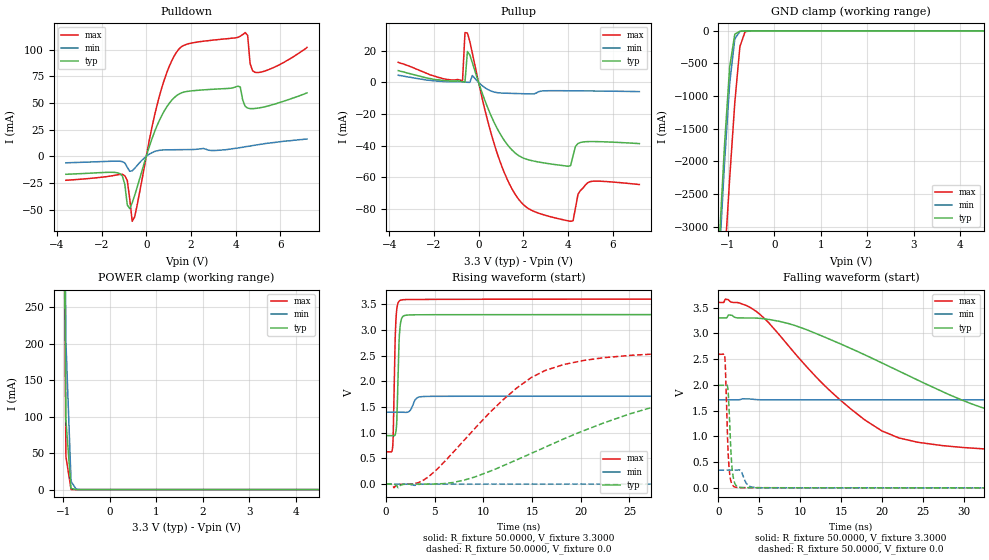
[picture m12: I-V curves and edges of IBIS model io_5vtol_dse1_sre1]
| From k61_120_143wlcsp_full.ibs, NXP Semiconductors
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[Model]  io_5vtol_dse1_sre1
|   Model io_5vtol_dse1_sre1
| Library cells for typ/min/max conditions are connected as defined below:
|  pad - External Pad
|  ipp_do - Core Input
|  ipp_obe - Output Buffer Enable
|  esd_boost - vdd_s_3v
|  esd_bus - vdd_s_3v
|  ipp_ame - vss_s_lv
|  ipp_dse - vdd_s_lv
|  ipp_ina40a_5vtol - NC
|  ipp_ina40b_5vtol - NC
|  ipp_ina_5vtol - NC
|  ipp_ina_mux_3v - NC
|  ipp_ind - NC
|  ipp_ind_3v - NC
|  ipp_pue - vss_s_lv
|  ipp_sre - vdd_s_lv
|  tie_3v - vdd_s_3v
|  tie_hi - vdd_s_lv
|  vbuf_3v - vdd_s_3v
|  vdd_bulk_lv - vdd_s_lv
|  vdd_s_3v - vdd_s_3v
|  vdd_s_lv - vdd_s_lv
|  vss_bulk - vss_s_3v
|  vss_s_3v - vss_s_3v
|  vss_s_lv - vss_s_lv
| All other pins connected to ground
Model_type I/O
Polarity   Non-Inverting
Enable   Active-High
Vinl =   1.1550V
Vinh =   2.3100V
Vmeas =  1.6500V
Cref =   25.0000pF
Rref =   50.0000
Vref =   0.0V
C_comp   2.8049pF   2.7887pF   2.9184pF
[Temperature Range]   25.0000   0.1250k   -40.0000
[Voltage Range]   3.3000V   1.7100V   3.6000V
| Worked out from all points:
|   slope of the pulldown table from 0 to 0.495 V, typ, clamps not added: 16.9 ohm
|   slope of the pullup table from 0 to 0.495 V, typ, clamps not added: 26 ohm
|   GND clamp passes 1 mA (typ) near -0.58 V on its own axis
|   POWER clamp passes 1 mA (typ) near -0.79 V on its own axis
|   rising waveform, R_fixture 50.0000, V_fixture 3.3000: 20-80 % time 211ps typ, 456ps min, 203ps max; typ from 0.944 V to 3.3 V
|   rising waveform, R_fixture 50.0000, V_fixture 0.0: 20-80 % time 17ns typ, 61.4ns min, 8.52ns max; typ from 0 V to 1.99 V
|   falling waveform, R_fixture 50.0000, V_fixture 3.3000: 20-80 % time 20.9ns typ, 77.8ns min, 11.6ns max; typ from 3.3 V to 0.944 V
|   falling waveform, R_fixture 50.0000, V_fixture 0.0: 20-80 % time 374ps typ, 586ps min, 338ps max; typ from 1.99 V to 0 V
[Pulldown]
|Voltage   I(typ)   I(min)   I(max)
-3.6V     -16.8mA    -6.04mA    -22.41mA
-960mV    -26.33mA   -6.164mA   -18.18mA
-850mV    -45.49mA   -10.23mA   -22.59mA
-630mV    -43.55mA   -13.55mA   -60.83mA
580mV     33.33mA    5.621mA    55.77mA
1.46V     58.28mA    6.233mA    100.4mA
4.1V      65.72mA    7.8mA      111.4mA
4.43V     46.8mA     9mA        115.9mA
4.54V     45.21mA    9.3mA      113.3mA
4.65V     44.72mA    9.6mA      86.87mA
4.98V     45.1mA     10.8mA     78.42mA
7.2V      59.4mA     16.2mA     102mA
[Pullup]
|Voltage   I(typ)   I(min)   I(max)
-3.6V     7.5mA      4.7mA      12.8mA
-720mV    488.7uA    342.9uA    955.4uA
-610mV    254.6uA    200.2uA    31.62mA
-500mV    19.62mA    91.27uA    31.26mA
930mV     -31.69mA   -6.615mA   -48.93mA
1.59V     -44.11mA   -6.982mA   -69.78mA
2.36V     -49.48mA   -7.293mA   -80.94mA
4.01V     -53.11mA   -5.27mA    -87.72mA
4.23V     -46.46mA   -5.29mA    -87.7mA
4.45V     -38.72mA   -5.32mA    -70.98mA
4.89V     -37.49mA   -5.38mA    -63.55mA
7.2V      -38.77mA   -5.81mA    -64.69mA
[GND_clamp]
|Voltage   I(typ)   I(min)   I(max)
-3.6V     -39.79A    -39.79A    -41.16A
-1.18V    -3.193A    -3.444A    -4.927A
-1.07V    -1.746A    -2.021A    -3.54A
-960mV    -554.7mA   -808.1mA   -2.265A
-850mV    -51.43mA   -125.2mA   -1.104A
-740mV    -5.185mA   -9.147mA   -242.4mA
-630mV    -1.474mA   -1.195mA   -14.98mA
-520mV    -384.8uA   -298.7uA   -1.148mA
7.2V      0A         0A         0A
[POWER_clamp]
|Voltage   I(typ)   I(min)   I(max)
-3.6V     45.62A     45.23A     45.93A
-1.05V    987.4mA    1.121A     927.4mA
-940mV    95.32mA    202.8mA    45.29mA
-830mV    1.645mA    11.46mA    218.1uA
-720mV    22.84uA    474.3uA    919.1nA
-610mV    316.6nA    19.24uA    4.178nA
7.2V      0A         0A         0A
[Ramp]
| variable   typ   min   max
dV/dt_r  1.1944/16.9607n   0.2054/61.3449n   1.5565/8.5237n
dV/dt_f  1.4137/20.9177n   0.1762/77.8009n   1.7829/11.5577n
R_load = 50.0000
[Rising Waveform]
R_fixture= 50.0000
V_fixture= 3.3000
V_fixture_min= 1.7100
V_fixture_max= 3.6000
|time   V(typ)   V(min)   V(max)
0s        943.7mV    1.399V     628.5mV
672.4ps   943.6mV    1.399V     727.5mV
730.8ps   943mV      1.399V     992.6mV
922ps     957.4mV    1.399V     2.802V
1.015ns   1.034V     1.399V     3.23V
1.094ns   1.235V     1.399V     3.41V
1.403ns   3.017V     1.399V     3.573V
1.878ns   3.28V      1.396V     3.591V
4.759ns   3.297V     1.708V     3.595V
250ns     3.3V       1.71V      3.6V
[Rising Waveform]
R_fixture= 50.0000
V_fixture= 0.0
V_fixture_min= 0.0
V_fixture_max= 0.0
|time   V(typ)   V(min)   V(max)
0s        463.5pV    70.75nV    297.1pV
806.7ps   -1.022mV   1.014uV    -74.28mV
4.371ns   -995.7uV   -309.5uV   144.3mV
11.9ns    345.9mV    -156.1uV   1.622V
16.34ns   719.7mV    -160.2uV   2.211V
27.48ns   1.502V     61.85uV    2.533V
35.99ns   1.792V     2.959mV    2.577V
58.34ns   1.964V     43.18mV    2.593V
139.8ns   1.991V     295.6mV    2.595V
250ns     1.991V     342.4mV    2.594V
[Falling Waveform]
R_fixture= 50.0000
V_fixture= 3.3000
V_fixture_min= 1.7100
V_fixture_max= 3.6000
|time   V(typ)   V(min)   V(max)
0s        3.3V       1.71V      3.6V
1.167ns   3.346V     1.71V      3.658V
4.627ns   3.297V     1.713V     3.425V
13.47ns   2.893V     1.71V      1.907V
19.95ns   2.426V     1.71V      1.106V
29.47ns   1.722V     1.71V      788.1mV
35.84ns   1.394V     1.709V     729.2mV
43.19ns   1.219V     1.705V     690.3mV
66.87ns   1.031V     1.674V     645.1mV
250ns     943.8mV    1.416V     628.5mV
[Falling Waveform]
R_fixture= 50.0000
V_fixture= 0.0
V_fixture_min= 0.0
V_fixture_max= 0.0
|time   V(typ)   V(min)   V(max)
0s        1.991V     344.3mV    2.594V
771.4ps   1.99V      344.3mV    2.547V
1.148ns   1.93V      344.3mV    794.2mV
1.405ns   1.102V     344.3mV    219.1mV
1.628ns   431.4mV    344.2mV    77.1mV
1.806ns   193.9mV    344.1mV    35mV
2.469ns   13.31mV    349mV      5.343mV
3.688ns   2.542mV    39.55mV    3.378mV
5.471ns   2.078mV    543.6uV    2.886mV
250ns     53.71nV    5.64uV     1.908nV
